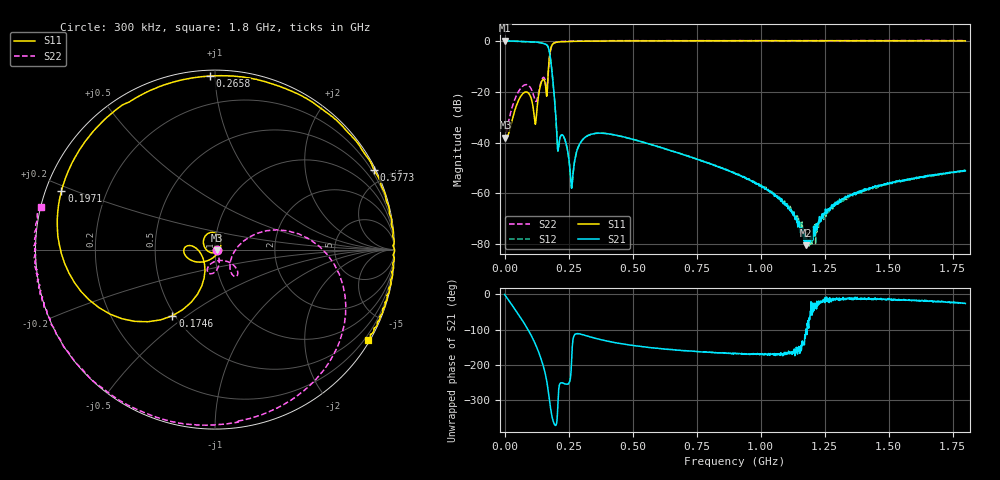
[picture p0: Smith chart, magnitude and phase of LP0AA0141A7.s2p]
!Agilent Technologies,E8358A,US40260310,A.06.04.32
!Agilent E8358A: A.06.04.32
!Date: Friday, October 18, 2019 00:04:17
!Correction: S11(Full 2 Port(1,2)) S21(Full 2 Port(1,2)) S12(Full 2 Port(1,2)) S22(Full 2 Port(1,2))
!S2P File: Measurements: S11, S21, S12, S22:
# Hz S  dB  R 50
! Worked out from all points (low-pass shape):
!   1601 points, 300 kHz to 1.8 GHz, reference 50 ohm
!   highest |S21| = -0.04 dB at 1.425 MHz (marker M1); lowest = -80.4 dB at 1.176 GHz (marker M2)
!   |S21| within 3 dB of the highest: start of sweep to 172.2 MHz
!   lowest |S11| = -38.1 dB at 3.674 MHz (marker M3), VSWR 1.03, Z = 51.2 - j0.418 ohm
!   |S11| at or under -10 dB: start of sweep to 172.3 MHz
!   |S22| runs from -39.0 to 0.1 dB; largest |S21 - S12| = 0.0082
!   S11 on the Smith chart (normalised r, x): 300 kHz: 1.03, +0.00; 174.6 MHz: 0.48, -0.44; 197.1 MHz: 0.05, +0.18; 265.8 MHz: 0.03, +0.97; 577.3 MHz: 0.08, +4.21; 1.8 GHz: 0.07, -3.66
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300000  -37.93 1.4  -0.05 -0.2  -0.11 -0.3  -39.03 -0.9
1424812  -37.92 -7.2  -0.04 -1.5  -0.11 -1.5  -38.74 -5.8
3674438  -38.09 -19.1  -0.05 -3.8  -0.11 -3.8  -37.99 -15.7
8.016169e7  -20.21 114.3  -0.33 -85.6  -0.37 -85.6  -17.33 -98.6
1.195301e8  -32.68 -17.2  -0.50 -139.3  -0.54 -139.2  -23.38 -93.0
1.352775e8  -20.00 -136.3  -0.69 -167.2  -0.73 -167.2  -19.14 -41.2
1.62273e8  -19.77 176.7  -1.48 124.3  -1.51 124.2  -17.70 -50.3
1.746459e8  -7.16 -122.8  -4.02 65.4  -4.06 65.3  -7.57 14.5
1.971422e8  -0.76 159.2  -25.39 -10.4  -25.40 -10.5  -0.75 -52.6
2.095151e8  -0.52 138.9  -43.04 70.7  -43.09 70.1  -0.45 -69.6
2.34261e8  -0.38 112.4  -38.38 107.1  -38.47 107.1  -0.22 -88.4
2.657558e8  -0.29 91.8  -54.45 -137.4  -54.48 -136.6  -0.10 -104.3
3.006249e8  -0.21 76.3  -39.44 -113.0  -39.44 -113.2  -0.08 -115.8
5.773288e8  -0.08 26.7  -40.93 -151.2  -40.91 -151.4  0.01 -151.5
6.009499e8  -0.05 24.7  -41.70 -152.7  -41.70 -152.9  -0.02 -153.1
9.0015e8  -0.07 4.5  -52.14 -167.6  -51.97 -165.5  0.04 -165.4
1.073371e9  -0.01 -3.7  -61.92 -170.4  -61.47 -167.7  -0.02 -170.3
1.175729e9  -0.03 -7.6  -80.40 -114.0  -79.06 -120.5  0.04 -173.3
1.200475e9  -0.00 -8.9  -77.21 -47.9  -79.92 -51.3  -0.01 -173.7
1.293834e9  -0.06 -12.4  -63.59 -14.1  -63.66 -15.7  0.04 -175.8
1.5008e9  -0.06 -19.7  -56.06 -11.1  -56.41 -17.4  0.07 178.9
1.8e9  -0.09 -30.6  -51.12 -25.6  -50.95 -26.0  0.00 166.2
